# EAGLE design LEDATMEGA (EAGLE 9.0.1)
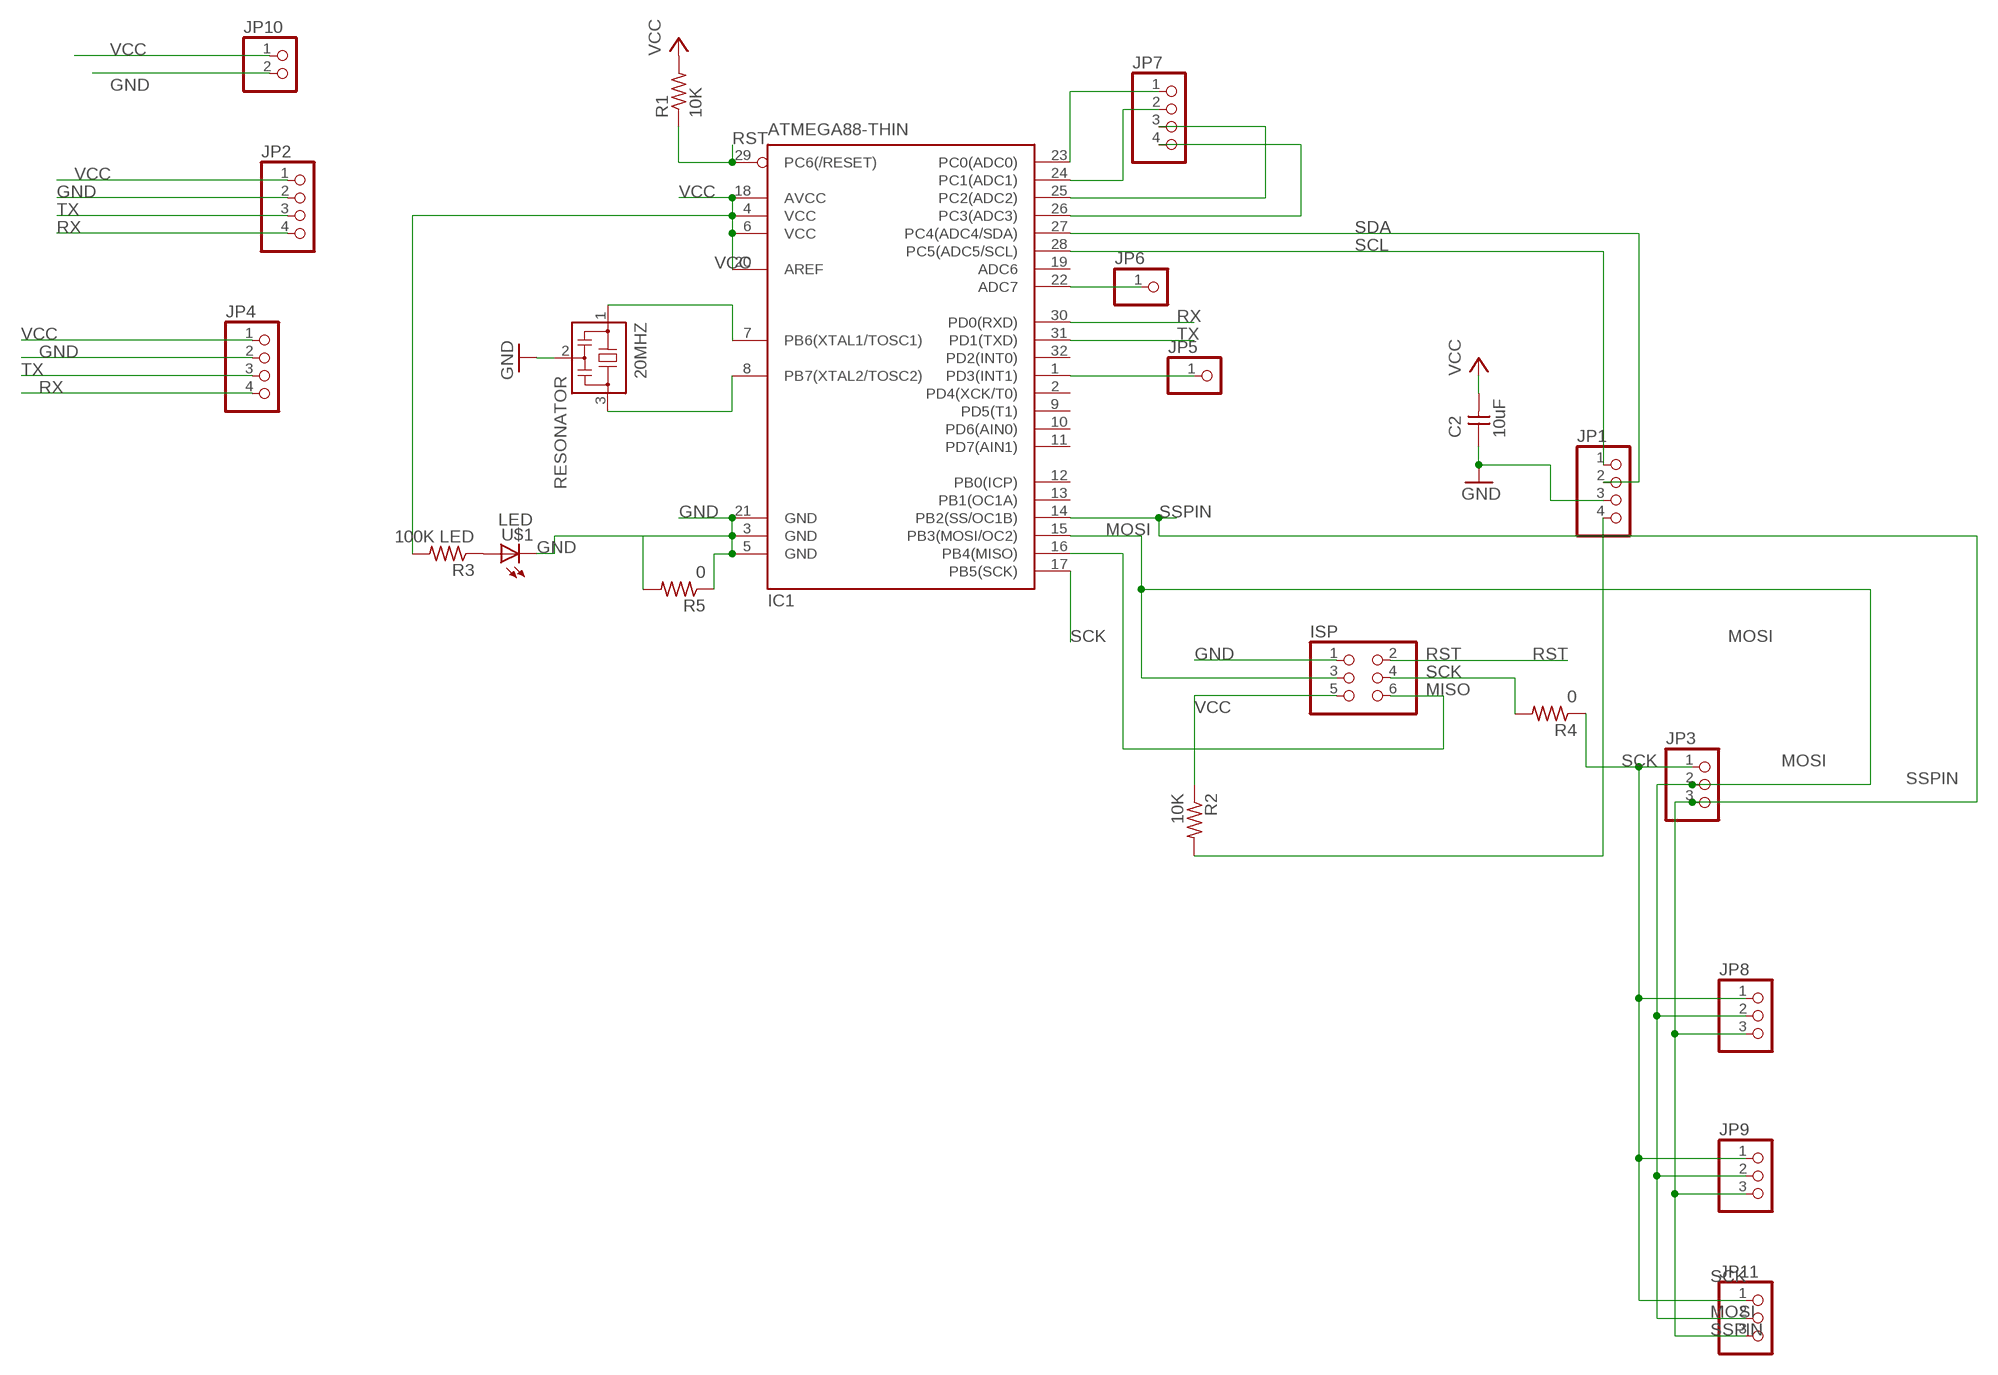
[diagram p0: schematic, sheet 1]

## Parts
20MHZ  RESONATOR  [EFOBM]
C2  10uF  CAP-UNPOLARIZEDFAB  [C1206FAB]
IC1  ATMEGA88-THIN  [TQFP32-08THIN]
ISP  PINHD-2X3-SMD  [2X03SMD]
JP1  PINHD-1X4  [1X04]
JP2  PINHD-1X4  [1X04]
JP3  PINHD-1X3CB  [1X03-CLEANBIG]
JP4  PINHD-1X4  [1X04]
JP5  PINHD-1X1  [1X01]
JP6  PINHD-1X1  [1X01]
JP7  PINHD-1X4  [1X04]
JP8  PINHD-1X3CB  [1X03-CLEANBIG]
JP9  PINHD-1X3CB  [1X03-CLEANBIG]
JP10  PINHD-1X2  [1X02]
JP11  PINHD-1X3CB  [1X03-CLEANBIG]
R1  10K  RES-US1206FAB  [R1206FAB]
R2  10K  RES-US1206FAB  [R1206FAB]
R3  100K LED  RES-US1206FAB  [R1206FAB]
R4  0  RES-US1206FAB  [R1206FAB]
R5  0  RES-US1206FAB  [R1206FAB]
U$1  LED  [LED1206]

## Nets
GND: 20MHZ.2 C2.1 IC1.3(GND) IC1.5(GND) IC1.21(GND) ISP.1 JP1.3 JP2.2 JP4.2 JP10.2 R5.1 R5.2 U$1.2(C)
MISO: IC1.16(PB4(MISO)) ISP.6
MOSI: IC1.15(PB3(MOSI/OC2)) ISP.3 JP3.2 JP8.2 JP9.2 JP11.2
N$1: JP1.4 R2.2
N$2: 20MHZ.1 IC1.7(PB6(XTAL1/TOSC1))
N$3: 20MHZ.3 IC1.8(PB7(XTAL2/TOSC2))
N$4: R3.1 U$1.1(A)
N$7: IC1.1(PD3(INT1)) JP5.1
N$8: IC1.22(ADC7) JP6.1
N$9: IC1.23(PC0(ADC0)) JP7.1
N$10: IC1.24(PC1(ADC1)) JP7.2
N$11: IC1.25(PC2(ADC2)) JP7.3
N$12: IC1.26(PC3(ADC3)) JP7.4
RST: IC1.29(PC6(/RESET)) ISP.2 R1.1
RX: IC1.30(PD0(RXD)) JP2.4 JP4.4
SCK: IC1.17(PB5(SCK)) ISP.4 JP3.1 JP8.1 JP9.1 JP11.1 R4.1 R4.2
SCL: IC1.28(PC5(ADC5/SCL)) JP1.1
SDA: IC1.27(PC4(ADC4/SDA)) JP1.2
SSPIN: IC1.14(PB2(SS/OC1B)) JP3.3 JP8.3 JP9.3 JP11.3
TX: IC1.31(PD1(TXD)) JP2.3 JP4.3
VCC: C2.2 IC1.4(VCC) IC1.6(VCC) IC1.18(AVCC) IC1.20(AREF) ISP.5 JP2.1 JP4.1 JP10.1 R1.2 R2.1 R3.2
Unconnected: IC1.2(PD4(XCK/T0)) IC1.9(PD5(T1)) IC1.10(PD6(AIN0)) IC1.11(PD7(AIN1)) IC1.12(PB0(ICP)) IC1.13(PB1(OC1A)) IC1.19(ADC6) IC1.32(PD2(INT0))

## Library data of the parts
20MHZ = fab:RESONATOR
C2 = fab:CAP-UNPOLARIZED
IC1 = fab:ATMEGA88-THIN
ISP = fab:PINHD-2X3-SMD: PIN HEADER
JP1 JP2 JP4 JP7 = pinhead:PINHD-1X4: PIN HEADER
JP3 JP8 JP9 JP11 = adafruit:PINHD-1X3: PIN HEADER
JP5 JP6 = pinhead:PINHD-1X1: PIN HEADER
JP10 = pinhead:PINHD-1X2: PIN HEADER
R1-R5 = fab:RES-US: Resistor (US Symbol)
U$1 = fab:LED: LED

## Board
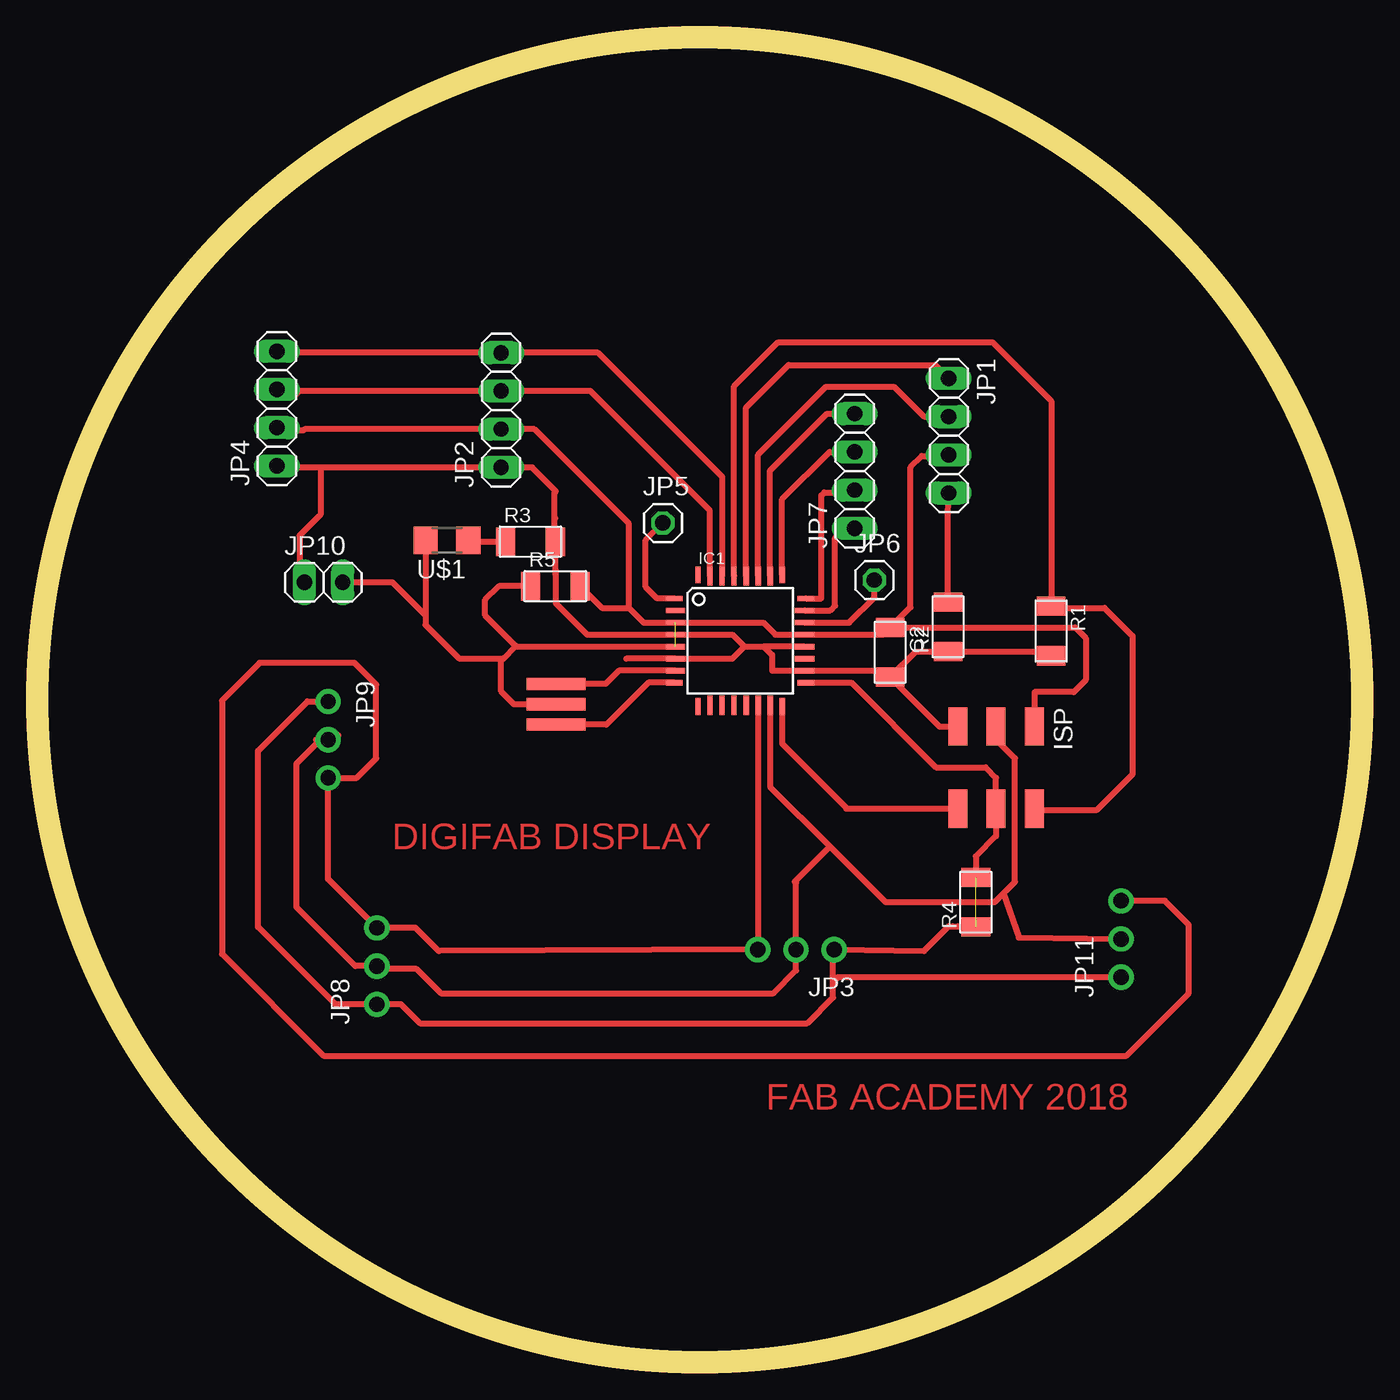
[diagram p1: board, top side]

Size 88 x 88 mm. Coordinates in mm from the lower left corner, seen from the top.
Outline: circle at 44,44 radius 44
Copper layers (1*16): Top 0.035mm / dielectric 1.5mm / Bottom 0.035mm
Design rules "default *": minimum track width 16mil, minimum drill 0.35mm, track to track 16mil, track to pad 16mil, pad to pad 16mil, via to via 16mil, smd to smd 16mil, copper to edge 40mil, drill to drill 6mil, minimum pad ring 10mil, minimum via ring 8mil, stop-mask expansion 4mil, vias tented up to drill 0mil, thermal gap 10mil

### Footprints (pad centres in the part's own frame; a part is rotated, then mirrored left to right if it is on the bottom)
EFOBM = smd 0.8 x 3.9: 1 -1.35,0; 2 0,0; 3 1.35,0
C1206FAB = smd 1.27 x 1.905: 1 -1.651,0; 2 1.651,0
TQFP32-08THIN = smd 1.118 x 0.356: 1 -4.369,2.8; 8 -4.369,-2.8; 17 4.369,-2.8; 24 4.369,2.8 | smd 1.27 x 0.356: 2 -4.293,2; 3 -4.293,1.2; 4 -4.293,0.4; 5 -4.293,-0.4; 6 -4.293,-1.2; 7 -4.293,-2; 18 4.293,-2; 19 4.293,-1.2; 20 4.293,-0.4; 21 4.293,0.4; 22 4.293,1.2; 23 4.293,2 | smd 0.356 x 1.118: 9 -2.8,-4.369; 16 2.8,-4.369; 25 2.8,4.369; 32 -2.8,4.369 | smd 0.356 x 1.27: 10 -2,-4.293; 14 1.2,-4.293; 15 2,-4.293; 26 2,4.293; 27 1.2,4.293; 31 -2,4.293 | smd 0.35 x 1.27: 11 -1.2,-4.293; 12 -0.4,-4.293; 13 0.4,-4.293; 28 0.4,4.293; 29 -0.4,4.293; 30 -1.2,4.293
2X03SMD = smd 2.54 x 1.27: 1 -2.54,2.54; 2 2.92,2.54; 3 -2.54,0; 4 2.92,0; 5 -2.54,-2.54; 6 2.92,-2.54
1X04 = drill 1.016 long: 1 -3.81,0; 2 -1.27,0; 3 1.27,0; 4 3.81,0
1X03-CLEANBIG = drill 1.016 pad 1.676: 1 -2.54,0; 2 0,0; 3 2.54,0
1X01 = drill 1.016 octagon: 1 0,0
1X02 = drill 1.016 long: 1 -1.27,0; 2 1.27,0
R1206FAB = smd 1.27 x 1.905: 1 -1.651,0; 2 1.651,0
LED1206 = smd 1.6 x 1.803: 1 -1.422,0; 2 1.422,0

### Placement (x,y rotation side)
20MHZ  34.45,43.7 270 top
C2  56.65,47.15 270 top
IC1  46.68,47.93 0 top
ISP  63.69,39.68 270 top
JP1  60.55,61.55 270 top
JP2  30.8,63.25 90 top
JP3  50.4,27.4 180 top
JP4  15.9,63.35 90 top
JP5  41.55,55.75 0 top
JP6  55.6,51.95 0 top
JP7  54.3,59.2 90 top
JP8  22.55,26.3 90 top
JP9  19.3,41.35 270 top
JP10  19,51.8 0 top
JP11  72,28.1 90 top
R1  67.35,48.57 270 top
R2  60.5,48.85 90 top
R3  32.75,54.5 0 top
R4  62.35,30.55 90 top
R5  34.4,51.55 0 top
U$1  27.2,54.6 180 top

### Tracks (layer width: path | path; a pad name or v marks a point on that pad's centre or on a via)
GND  (1 unrouted)
  Top 0.406: C2.1 56.18,48.33 IC1.21 49.02,48.33 48.22,49.13 IC1.3 40.27,49.13 39.3,50.1 | C2.1 56.85,48.6 | C2.1 68.95,48.8 69.65,48.1 69.65,45.3 68.85,44.5 66.25,44.5 66.25,42.24 ISP.1 | 20MHZ.2 31.65,43.7 30.8,44.55 30.8,46.6 30.95,46.75 | 30.95,46.75 31.73,47.53 | 31.73,47.53 IC1.5 | JP4.2 16.08,61.9 17.65,61.9 17.73,61.98 JP2.2 33.02,61.98 39.3,55.7 39.3,50.1 | C2.1 58,50.15 58,59.45 58.75,60.2 60.63,60.2 | 61.35,60.2 60.63,60.2 | 60.63,60.2 JP1.3 | U$1.2 25.78,49.6 | 25.78,49.6 25.78,48.97 28,46.75 30.95,46.75 | 31.73,47.53 31.73,47.62 29.75,49.6 29.75,50.65 30.65,51.55 R5.1 | R5.2 37.5,50.1 39.3,50.1 | 25.78,49.6 23.58,51.8 JP10.2
MISO
  Top 0.406: IC1.16 49.48,41.08 53.74,36.82 53.74,36.76 ISP.6
MOSI
  Top 0.406: IC1.15 48.68,38.22 52.65,34.25 | ISP.3 63.69,41.36 64.95,40.1 64.95,31.9 64.18,31.12 | 52.65,34.25 50.32,31.92 50.4,31.84 JP3.2 50.4,26 48.9,24.5 26.8,24.5 25.2,26.1 22.75,26.1 JP8.2 21.1,26.3 17.2,30.2 17.2,39.75 18.8,41.35 | 52.65,34.25 56.35,30.55 63.6,30.55 64.18,31.12 | 19.8,41.55 20,41.65 19.7,41.35 JP9.2 18.8,41.35 | 64.18,31.12 65.2,28.2 JP11.2 | 18.5,41.35 18.8,41.35
N$1
  Top 0.406: R2.2 60.5,56.39 JP1.4
N$2
  Top 0.406: IC1.7 38.63,45.93 37.75,45.05 20MHZ.1
N$3
  Top 0.406: IC1.8 40.58,45.13 37.8,42.35 20MHZ.3
N$4
  Top 0.406: U$1.1 28.72,54.5 R3.1
N$7
  Top 0.406: IC1.1 41.17,50.73 40.4,51.5 40.4,54.6 JP5.1
N$8
  Top 0.406: IC1.22 53.93,49.13 55.6,50.8 JP6.1
N$9
  Top 0.406: IC1.23 52.68,49.93 53,50.25 53,54.75 53.64,55.39 JP7.1
N$10
  Top 0.406: IC1.24 52.08,50.73 52.08,57.57 52.28,57.77 54.14,57.77 JP7.2
N$11
  Top 0.406: IC1.25 49.48,57.33 52.62,60.47 JP7.3
N$12
  Top 0.406: IC1.26 48.68,59.23 52.46,63.01 JP7.4
RST
  Top 0.406: ISP.2 66.34,36.65 70.35,36.65 72.75,39.05 72.75,48.25 70.9,50.1 67.47,50.1 R1.1 67.35,63.85 63.45,67.75 49.2,67.75 46.28,64.83 IC1.29
RX
  Top 0.406: IC1.30 45.48,58.82 37.24,67.06 JP2.4 | JP2.4 | JP4.4 16,67.06 JP2.4
SCK  (1 unrouted)
  Top 0.406: IC1.17 54.07,45.13 59.7,39.5 63,39.5 63.69,38.81 ISP.4 63.69,34.94 62.35,33.6 R4.2 | 60.8,28.95 61.16,28.94 | 61.16,28.94 R4.1 | JP9.1 17.94,43.89 14.65,40.6 14.65,28.9 19.79,23.76 JP8.1 24.14,23.76 25.4,22.5 51.15,22.5 52.86,24.21 52.86,25.25 | 52.86,25.25 52.86,27.22 JP3.1 58.9,27.3 60.54,28.94 61.16,28.94 | 52.86,25.25 53.17,25.56 JP11.1
SCL
  Top 0.406: 59.21,65.3 JP1.1 59.66,66.25 49.9,66.25 47.08,63.43 IC1.28
SDA
  Top 0.406: IC1.27 47.88,60.28 52.4,64.8 56.9,64.8 58.88,62.82 JP1.2
SSPIN
  Top 0.406: JP11.3 74.91,30.64 76.5,29.05 76.5,24.5 72.35,20.35 19,20.35 12.25,27.1 12.25,43.95 14.75,46.45 21.05,46.45 22.5,45 22.5,40.1 21.21,38.81 JP9.3 19.3,32.09 JP8.3 25.11,28.84 26.65,27.3 JP3.3 47.88,27.32 IC1.14
TX
  Top 0.406: IC1.31 44.68,56.57 36.73,64.52 JP2.3 | 30.83,64.55 JP2.3 | JP2.3 17.37,64.52 17.1,64.25 16.27,64.25 JP4.3
VCC
  Top 0.406: C2.2 56.65,45.3 56.02,45.93 IC1.18 48.82,45.93 48.8,45.95 48.8,46.98 48.25,47.53 | 56.6,45.45 C2.2 | 46.97,47.53 48.25,47.53 | 46.97,47.53 46.17,48.33 IC1.4 36.52,48.33 34.43,50.42 34.43,52.6 | 46.97,47.53 46.17,46.73 IC1.6 39.12,46.73 | C2.2 59.93,42.22 ISP.5 | C2.2 58.35,47.2 R2.1 67.07,47.2 R1.2 | JP2.1 18.8,59.44 | 18.8,59.44 17.14,59.44 | 17.14,59.44 17,59.3 | 34.43,52.27 34.43,52.6 | 34.43,52.6 R3.2 34.35,56 | IC1.20 48.25,47.53 | JP4.1 16,59.44 17.14,59.44 | 34.35,56 34.4,56.05 | 32.41,59.44 JP2.1 | 34.35,56 34.35,57.75 34.45,57.85 32.86,59.44 JP2.1 | 18.8,59.44 18.8,56.3 17.4,54.9 17.4,52.13 JP10.1

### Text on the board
Top: DIGIFAB DISPLAY | FAB ACADEMY 2018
